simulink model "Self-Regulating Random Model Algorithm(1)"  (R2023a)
settings: Solver=VariableStepAuto  StartTime=0.0  StopTime=20  RelTol=1e-3
libraries: simulink x63, spspowerguiLib x1
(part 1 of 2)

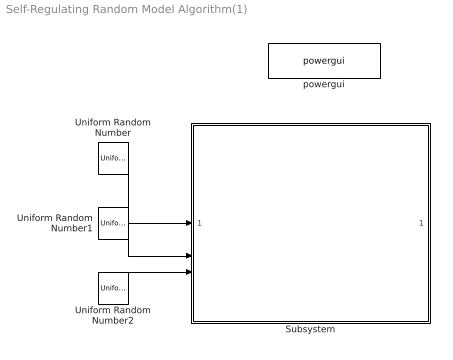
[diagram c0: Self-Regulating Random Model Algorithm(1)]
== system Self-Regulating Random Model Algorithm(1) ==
  Subsystem : Subsystem
  Uniform Random Number : UniformRandomNumber  Minimum=0  Seed=1111  SampleTime=1e-4
  Uniform Random Number1 : UniformRandomNumber  Minimum=0  Seed=3232  SampleTime=1e-4
  Uniform Random Number2 : UniformRandomNumber  Minimum=0  Seed=5566  SampleTime=1e-4
  powergui : spspowerguiLib/powergui  Priority=1  SimulationMode=Discrete  SampleTime=1e-4  frequency=60  Iterations=50  frequencyindice=0  Pbase=100e6  ErrMax=1e-4  UnitsV=kV  UnitsW=MW  buscounter=0  FunctionMessages=off  echomessages=off  EnableUseOfTLC=off  CurrentSourceSwitches=off  DisableSnubberDevices=off  DisableRonSwitches=off  DisableVfSwitches=off  DisplayEquations=off  AutomaticDiscreteSolvers=off  SolverType=Tustin  Interpol=off  ExternalGateDelay=off  methode=off  Ts=0  x0status=blocks  SPID=off  SwTol=0  HookPort=off  NonlinearTolerance=1e-4  nMaxIteration=100  ContinueOnMaxIteration=off  RestoreLinks=warning  ResistiveCurrentMeasurement=off  Frange=[0:2:500]  Ylog=off  Xlog=on  ShowGrid=off  save=off  variable=ZData  structure=sco_motor_wr  ZoomFFT=off  StartTime=4  cycles=75  DisplayStyle=5  fundamental=40  FreqAxis=off  MaxFrequency=300  frequencyindicesteady=1  RmsSteady=1  display=off
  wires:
  Uniform Random Number2/1 -> Subsystem/3(Random_num_add)
  Uniform Random Number1/1 -> Subsystem/2(Random_num_adc)
  Uniform Random Number/1 -> Subsystem/1(Random_num_select)
  Subsystem/1(injection_num) -> ?  "inj_num"

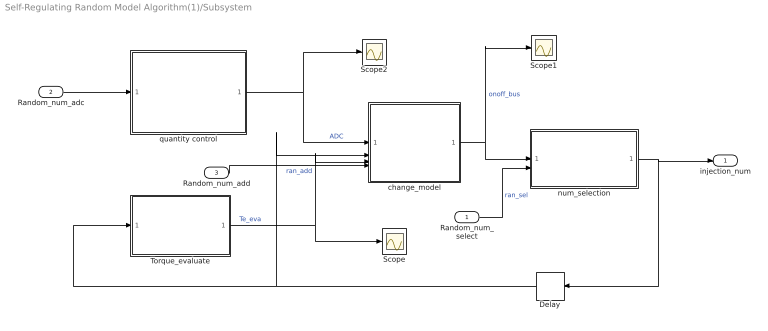
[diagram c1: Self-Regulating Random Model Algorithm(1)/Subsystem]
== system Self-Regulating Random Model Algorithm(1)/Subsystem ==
  Random_num_select : Inport
  Random_num_adc : Inport  Port=2
  Random_num_add : Inport  Port=3
  Delay : Delay  DelayLength=1  InitialCondition=2
  Scope : Scope
  Scope1 : Scope
  Scope2 : Scope
  Torque_evaluate : Subsystem
  change_model : Subsystem
  num_selection : Subsystem
  quantity control : Subsystem
  injection_num : Outport
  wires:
  change_model/1(on/off_signal) -> Scope1/1, num_selection/1(on/off_signal)  "onoff_bus"
  Torque_evaluate/1(Te_eva) -> change_model/3(Te_eva), Scope/1  "Te_eva"
  quantity control/1(A/D/C_operation) -> Scope2/1, change_model/1(A/D/C)  "ADC"
  Delay/1 -> change_model/2(last_num), Torque_evaluate/1(injection_num)
  Random_num_select/1 -> num_selection/2(Random_num)  "ran_sel"
  num_selection/1(injection_num) -> injection_num/1, Delay/1
  Random_num_adc/1 -> quantity control/1(Random_num)
  Random_num_add/1 -> change_model/4(Random_num)  "ran_add"

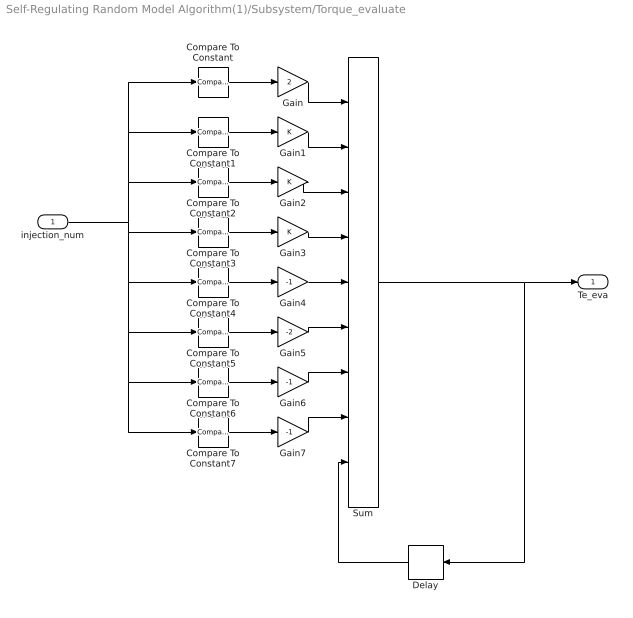
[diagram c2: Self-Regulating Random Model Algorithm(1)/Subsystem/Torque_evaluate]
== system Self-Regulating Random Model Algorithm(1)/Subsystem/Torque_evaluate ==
  injection_num : Inport
  Compare To Constant : simulink/Logic and Bit Operations/Compare To Constant  relop===  const=1  OutDataTypeStr=boolean
  Compare To Constant1 : simulink/Logic and Bit Operations/Compare To Constant  relop===  const=2  OutDataTypeStr=boolean
  Compare To Constant2 : simulink/Logic and Bit Operations/Compare To Constant  relop===  const=8  OutDataTypeStr=boolean
  Compare To Constant3 : simulink/Logic and Bit Operations/Compare To Constant  relop===  const=9  OutDataTypeStr=boolean
  Compare To Constant4 : simulink/Logic and Bit Operations/Compare To Constant  relop===  const=4  OutDataTypeStr=boolean
  Compare To Constant5 : simulink/Logic and Bit Operations/Compare To Constant  relop===  const=5  OutDataTypeStr=boolean
  Compare To Constant6 : simulink/Logic and Bit Operations/Compare To Constant  relop===  const=6  OutDataTypeStr=boolean
  Compare To Constant7 : simulink/Logic and Bit Operations/Compare To Constant  relop===  const=11  OutDataTypeStr=boolean
  Delay : Delay  DelayLength=1  InitialCondition=0
  Gain : Gain  Gain=2  OutDataTypeStr=single
  Gain1 : Gain  OutDataTypeStr=single
  Gain2 : Gain  OutDataTypeStr=single
  Gain3 : Gain  OutDataTypeStr=single
  Gain4 : Gain  Gain=-1  OutDataTypeStr=single
  Gain5 : Gain  Gain=-2  OutDataTypeStr=single
  Gain6 : Gain  Gain=-1  OutDataTypeStr=single
  Gain7 : Gain  Gain=-1  OutDataTypeStr=single
  Sum : Sum  Inputs=+++++++++
  Te_eva : Outport
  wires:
  injection_num/1 -> Compare To Constant5/1, Compare To Constant6/1, Compare To Constant7/1, Compare To Constant4/1, Compare To Constant3/1, Compare To Constant1/1, Compare To Constant/1, Compare To Constant2/1
  Compare To Constant/1 -> Gain/1
  Compare To Constant1/1 -> Gain1/1
  Compare To Constant2/1 -> Gain2/1
  Compare To Constant3/1 -> Gain3/1
  Compare To Constant4/1 -> Gain4/1
  Compare To Constant5/1 -> Gain5/1
  Gain5/1 -> Sum/6
  Gain4/1 -> Sum/5
  Gain3/1 -> Sum/4
  Gain2/1 -> Sum/3
  Gain1/1 -> Sum/2
  Gain/1 -> Sum/1
  Sum/1 -> Delay/1, Te_eva/1
  Delay/1 -> Sum/9
  Compare To Constant7/1 -> Gain7/1
  Gain6/1 -> Sum/7
  Gain7/1 -> Sum/8
  Compare To Constant6/1 -> Gain6/1

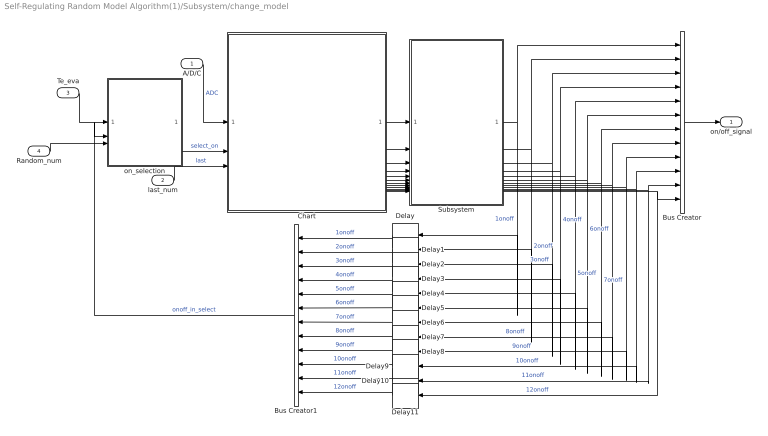
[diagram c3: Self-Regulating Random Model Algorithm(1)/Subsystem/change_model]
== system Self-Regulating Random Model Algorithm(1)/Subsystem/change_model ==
  A/D/C : Inport
  last_num : Inport  Port=2
  Te_eva : Inport  Port=3
  Random_num : Inport  Port=4
  Bus Creator : BusCreator  Inputs=12
  Bus Creator1 : BusCreator  Inputs=12
  Chart : Stateflow chart  TreatAsAtomicUnit=on
  Delay{,1,3..5,7} (6 alike) : Delay  DelayLength=1  InitialCondition=1
  Delay{2,6,8..11} (6 alike) : Delay  DelayLength=1  InitialCondition=0
  Subsystem : Subsystem
  on_selection : Subsystem
  on/off_signal : Outport
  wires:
  Subsystem/5(Condition5) -> Delay4/1, Bus Creator/5  "5onoff"
  Subsystem/6(Condition6) -> Delay5/1, Bus Creator/6  "6onoff"
  Subsystem/7(Condition7) -> Delay6/1, Bus Creator/7  "7onoff"
  Subsystem/8(Condition8) -> Bus Creator/8, Delay7/1  "8onoff"
  Subsystem/9(Condition9) -> Delay8/1, Bus Creator/9  "9onoff"
  Subsystem/10(Condition10) -> Delay9/1, Bus Creator/10  "10onoff"
  Subsystem/11(Condition11) -> Bus Creator/11, Delay10/1  "11onoff"
  Subsystem/12(Condition12) -> Bus Creator/12, Delay11/1  "12onoff"
  Subsystem/1(Condition1) -> Bus Creator/1, Delay/1  "1onoff"
  Subsystem/2(Condition2) -> Bus Creator/2, Delay1/1  "2onoff"
  Subsystem/3(Condition3) -> Delay2/1, Bus Creator/3  "3onoff"
  Subsystem/4(Condition4) -> Delay3/1, Bus Creator/4  "4onoff"
  Bus Creator/1 -> on/off_signal/1
  Te_eva/1 -> on_selection/1(Te_eva)
  Random_num/1 -> on_selection/3(Random_num2)
  Chart/1(Trigger1) -> Subsystem/1(Trigger1)
  Chart/2(Trigger2) -> Subsystem/2(Trigger2)
  Chart/3(Trigger3) -> Subsystem/3(Trigger3)
  Chart/4(Trigger4) -> Subsystem/4(Trigger4)
  Chart/5(Trigger5) -> Subsystem/5(Trigger5)
  Chart/6(Trigger6) -> Subsystem/6(Trigger6)
  Chart/7(Trigger7) -> Subsystem/7(Trigger7)
  Chart/8(Trigger8) -> Subsystem/8(Trigger8)
  Chart/9(Trigger9) -> Subsystem/9(Trigger9)
  Chart/10(Trigger10) -> Subsystem/10(Trigger10)
  Chart/11(Trigger11) -> Subsystem/11(Trigger11)
  Chart/12(Trigger12) -> Subsystem/12(Trigger12)
  on_selection/1(select_on_num) -> Chart/2(select_on_num)  "select_on"
  last_num/1 -> Chart/3(last_num)  "last"
  A/D/C/1 -> Chart/1(A_D_C)  "ADC"
  Delay7/1 -> Bus Creator1/8  "8onoff"
  Delay10/1 -> Bus Creator1/11  "11onoff"
  Delay2/1 -> Bus Creator1/3  "3onoff"
  Delay5/1 -> Bus Creator1/6  "6onoff"
  Delay4/1 -> Bus Creator1/5  "5onoff"
  Delay6/1 -> Bus Creator1/7  "7onoff"
  Delay/1 -> Bus Creator1/1  "1onoff"
  Delay11/1 -> Bus Creator1/12  "12onoff"
  Delay1/1 -> Bus Creator1/2  "2onoff"
  Delay9/1 -> Bus Creator1/10  "10onoff"
  Delay3/1 -> Bus Creator1/4  "4onoff"
  Delay8/1 -> Bus Creator1/9  "9onoff"
  Bus Creator1/1 -> on_selection/2(on/off_bus2)  "onoff_in_select"

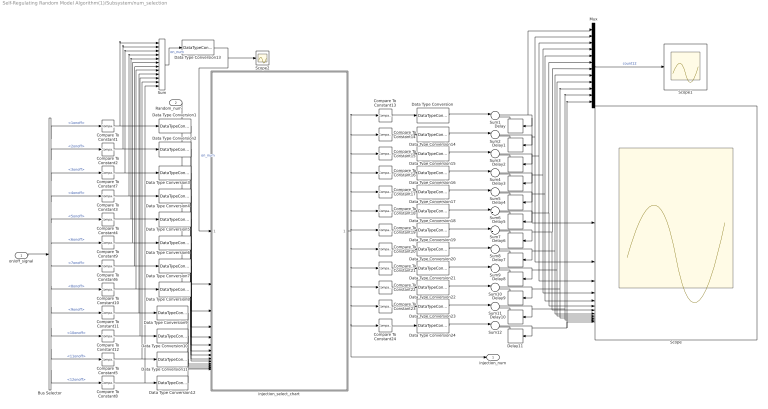
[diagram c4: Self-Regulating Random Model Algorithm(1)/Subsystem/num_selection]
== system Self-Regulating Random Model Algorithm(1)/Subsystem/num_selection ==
  on/off_signal : Inport
  Random_num : Inport  Port=2
  Bus Selector : BusSelector  OutputSignals=1onoff,2onoff,3onoff,4onoff,5onoff,6onoff,7onoff,8onoff,9onoff,10onoff,11onoff,12onoff
  Compare To Constant{1..12} (12 alike) : simulink/Logic and Bit Operations/Compare To Constant  relop===  const=1  OutDataTypeStr=boolean
  Compare To Constant13 : simulink/Logic and Bit Operations/Compare To Constant  relop===  const=1  OutDataTypeStr=uint8
  Compare To Constant14 : simulink/Logic and Bit Operations/Compare To Constant  relop===  const=2  OutDataTypeStr=uint8
  Compare To Constant15 : simulink/Logic and Bit Operations/Compare To Constant  relop===  const=3  OutDataTypeStr=uint8
  Compare To Constant16 : simulink/Logic and Bit Operations/Compare To Constant  relop===  const=4  OutDataTypeStr=uint8
  Compare To Constant17 : simulink/Logic and Bit Operations/Compare To Constant  relop===  const=5  OutDataTypeStr=uint8
  Compare To Constant18 : simulink/Logic and Bit Operations/Compare To Constant  relop===  const=6  OutDataTypeStr=uint8
  Compare To Constant19 : simulink/Logic and Bit Operations/Compare To Constant  relop===  const=7  OutDataTypeStr=uint8
  Compare To Constant20 : simulink/Logic and Bit Operations/Compare To Constant  relop===  const=8  OutDataTypeStr=uint8
  Compare To Constant21 : simulink/Logic and Bit Operations/Compare To Constant  relop===  const=9  OutDataTypeStr=uint8
  Compare To Constant22 : simulink/Logic and Bit Operations/Compare To Constant  relop===  const=10  OutDataTypeStr=uint8
  Compare To Constant23 : simulink/Logic and Bit Operations/Compare To Constant  relop===  const=11  OutDataTypeStr=uint8
  Compare To Constant24 : simulink/Logic and Bit Operations/Compare To Constant  relop===  const=12  OutDataTypeStr=uint8
  Data Type Conversion{,13..24} (13 alike) : DataTypeConversion  OutDataTypeStr=single
  Data Type Conversion{1..12} (12 alike) : DataTypeConversion  OutDataTypeStr=uint8
  Delay{,1..11} (12 alike) : Delay  DelayLength=1  InitialCondition=0
  Mux : Mux  Inputs=12
  Scope : Scope  NumInputPorts=12
  Scope1 : Scope
  Scope2 : Scope
  Sum : Sum  Inputs=++++++++++++
  Sum{1..12} (12 alike) : Sum  Inputs=|++
  injection_select_chart : Stateflow chart  TreatAsAtomicUnit=on
  injection_num : Outport
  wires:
  Bus Selector/11 -> Compare To Constant5/1  "<11onoff>"
  Bus Selector/7 -> Compare To Constant6/1  "<7onoff>"
  Bus Selector/3 -> Compare To Constant7/1  "<3onoff>"
  Bus Selector/2 -> Compare To Constant2/1  "<2onoff>"
  on/off_signal/1 -> Bus Selector/1
  Bus Selector/6 -> Compare To Constant9/1  "<6onoff>"
  Bus Selector/5 -> Compare To Constant4/1  "<5onoff>"
  Bus Selector/1 -> Compare To Constant1/1  "<1onoff>"
  Bus Selector/8 -> Compare To Constant10/1  "<8onoff>"
  Bus Selector/9 -> Compare To Constant11/1  "<9onoff>"
  Bus Selector/4 -> Compare To Constant3/1  "<4onoff>"
  Bus Selector/10 -> Compare To Constant12/1  "<10onoff>"
  Bus Selector/12 -> Compare To Constant8/1  "<12onoff>"
  Compare To Constant1/1 -> Sum/1, Data Type Conversion1/1
  Compare To Constant2/1 -> Data Type Conversion2/1, Sum/2
  Compare To Constant3/1 -> Sum/4, Data Type Conversion4/1
  Compare To Constant9/1 -> Sum/6, Data Type Conversion6/1
  Compare To Constant4/1 -> Sum/5, Data Type Conversion5/1
  Compare To Constant10/1 -> Sum/8, Data Type Conversion8/1
  Compare To Constant12/1 -> Sum/10, Data Type Conversion10/1
  Compare To Constant11/1 -> Sum/9, Data Type Conversion9/1
  Compare To Constant8/1 -> Sum/12, Data Type Conversion12/1
  Compare To Constant7/1 -> Sum/3, Data Type Conversion3/1
  Compare To Constant6/1 -> Sum/7, Data Type Conversion7/1
  Compare To Constant5/1 -> Sum/11, Data Type Conversion11/1
  Random_num/1 -> injection_select_chart/2(Random_num)
  Data Type Conversion13/1 -> Scope2/1, injection_select_chart/1(On_num)  "on_num"
  injection_select_chart/1(Injection_num) -> Compare To Constant19/1, Compare To Constant18/1, Compare To Constant17/1, Compare To Constant16/1, Compare To Constant15/1, Compare To Constant14/1, Compare To Constant13/1, Compare To Constant20/1, Compare To Constant21/1, Compare To Constant22/1, Compare To Constant23/1, Compare To Constant24/1, injection_num/1
  Data Type Conversion1/1 -> injection_select_chart/3(oo1)
  Data Type Conversion2/1 -> injection_select_chart/4(oo2)
  Data Type Conversion3/1 -> injection_select_chart/5(oo3)
  Data Type Conversion4/1 -> injection_select_chart/6(oo4)
  Data Type Conversion5/1 -> injection_select_chart/7(oo5)
  Data Type Conversion6/1 -> injection_select_chart/8(oo6)
  Data Type Conversion7/1 -> injection_select_chart/9(oo7)
  Data Type Conversion8/1 -> injection_select_chart/10(oo8)
  Data Type Conversion9/1 -> injection_select_chart/11(oo9)
  Data Type Conversion10/1 -> injection_select_chart/12(oo10)
  Data Type Conversion11/1 -> injection_select_chart/13(oo11)
  Data Type Conversion12/1 -> injection_select_chart/14(oo12)
  Sum/1 -> Data Type Conversion13/1  "on_num"
  Sum1/1 -> Mux/1, Delay/1, Scope/1
  Compare To Constant13/1 -> Data Type Conversion/1
  Delay/1 -> Sum1/2
  Delay1/1 -> Sum2/2
  Sum2/1 -> Delay1/1, Mux/2, Scope/2
  Compare To Constant14/1 -> Data Type Conversion14/1
  Delay2/1 -> Sum3/2
  Sum3/1 -> Delay2/1, Mux/3, Scope/3
  Compare To Constant15/1 -> Data Type Conversion15/1
  Delay3/1 -> Sum4/2
  Sum4/1 -> Delay3/1, Mux/4, Scope/4
  Compare To Constant16/1 -> Data Type Conversion16/1
  Delay4/1 -> Sum5/2
  Sum5/1 -> Delay4/1, Mux/5, Scope/5
  Compare To Constant17/1 -> Data Type Conversion17/1
  Delay5/1 -> Sum6/2
  Sum6/1 -> Delay5/1, Mux/6, Scope/6
  Compare To Constant18/1 -> Data Type Conversion18/1
  Delay6/1 -> Sum7/2
  Sum7/1 -> Delay6/1, Mux/7, Scope/7
  Compare To Constant19/1 -> Data Type Conversion19/1
  Delay7/1 -> Sum8/2
  Sum8/1 -> Delay7/1, Mux/8, Scope/8
  Compare To Constant20/1 -> Data Type Conversion20/1
  Delay8/1 -> Sum9/2
  Sum9/1 -> Delay8/1, Mux/9, Scope/9
  Compare To Constant21/1 -> Data Type Conversion21/1
  Delay9/1 -> Sum10/2
  Sum10/1 -> Delay9/1, Mux/10, Scope/10
  Compare To Constant22/1 -> Data Type Conversion22/1
  Delay10/1 -> Sum11/2
  Sum11/1 -> Delay10/1, Mux/11, Scope/11
  Compare To Constant23/1 -> Data Type Conversion23/1
  Delay11/1 -> Sum12/2
  Sum12/1 -> Delay11/1, Mux/12, Scope/12
  Compare To Constant24/1 -> Data Type Conversion24/1
  Data Type Conversion/1 -> Sum1/1
  Data Type Conversion14/1 -> Sum2/1
  Data Type Conversion15/1 -> Sum3/1
  Data Type Conversion16/1 -> Sum4/1
  Data Type Conversion17/1 -> Sum5/1
  Data Type Conversion18/1 -> Sum6/1
  Data Type Conversion19/1 -> Sum7/1
  Data Type Conversion20/1 -> Sum8/1
  Data Type Conversion21/1 -> Sum9/1
  Data Type Conversion22/1 -> Sum10/1
  Data Type Conversion23/1 -> Sum11/1
  Data Type Conversion24/1 -> Sum12/1
  Mux/1 -> Scope1/1  "count12"

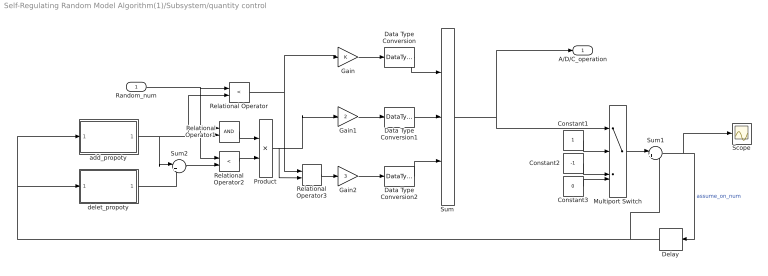
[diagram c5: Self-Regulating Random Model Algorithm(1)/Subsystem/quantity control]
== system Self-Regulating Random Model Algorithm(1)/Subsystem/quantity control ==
  Random_num : Inport
  Constant1 : Constant  OutDataTypeStr=single
  Constant2 : Constant  Value=-1  OutDataTypeStr=single
  Constant3 : Constant  Value=0  OutDataTypeStr=single
  Data Type Conversion : DataTypeConversion  OutDataTypeStr=uint16
  Data Type Conversion1 : DataTypeConversion  OutDataTypeStr=uint16
  Data Type Conversion2 : DataTypeConversion  OutDataTypeStr=uint16
  Delay : Delay  DelayLength=1  InitialCondition=7
  Gain : Gain
  Gain1 : Gain  Gain=2
  Gain2 : Gain  Gain=3
  Multiport Switch : MultiPortSwitch  DiagnosticForDefault=None
  Product : Product
  Relational Operator : RelationalOperator  Operator=<  OutDataTypeStr=boolean
  Relational Operator1 : RelationalOperator  OutDataTypeStr=boolean
  Relational Operator2 : RelationalOperator  Operator=<  OutDataTypeStr=boolean
  Relational Operator3 : RelationalOperator  Operator===  OutDataTypeStr=boolean
  Scope : Scope
  Sum : Sum  Inputs=+++
  Sum1 : Sum  Inputs=|++
  Sum2 : Sum  Inputs=|++
  add_propoty : Subsystem
  delet_propoty : Subsystem
  A/D/C_operation : Outport
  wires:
  Delay/1 -> Sum1/2, delet_propoty/1(Qtt), add_propoty/1(Qtt)
  Gain2/1 -> Data Type Conversion2/1
  Data Type Conversion2/1 -> Sum/3
  Data Type Conversion1/1 -> Sum/2
  Data Type Conversion/1 -> Sum/1
  Gain1/1 -> Data Type Conversion1/1
  Gain/1 -> Data Type Conversion/1
  Random_num/1 -> Relational Operator2/1, Relational Operator1/1, Relational Operator/1
  add_propoty/1(Ppt) -> Sum2/1, Relational Operator1/2, Relational Operator/2
  Relational Operator/1 -> Relational Operator3/1, Gain/1
  Relational Operator1/1 -> Product/1
  Relational Operator2/1 -> Product/2
  Product/1 -> Relational Operator3/2, Gain1/1
  Relational Operator3/1 -> Gain2/1
  Constant1/1 -> Multiport Switch/2
  Constant2/1 -> Multiport Switch/3
  Constant3/1 -> Multiport Switch/4
  Multiport Switch/1 -> Sum1/1
  Sum1/1 -> Scope/1, Delay/1  "assume_on_num"
  Sum2/1 -> Relational Operator2/2
  delet_propoty/1(Ppt) -> Sum2/2
  Sum/1 -> A/D/C_operation/1, Multiport Switch/1

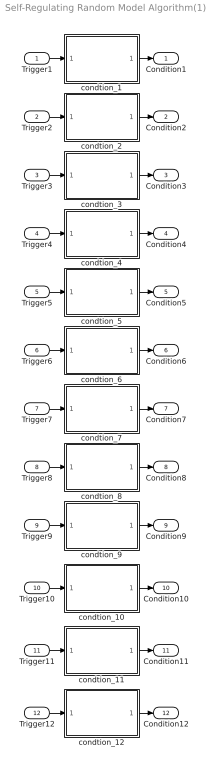
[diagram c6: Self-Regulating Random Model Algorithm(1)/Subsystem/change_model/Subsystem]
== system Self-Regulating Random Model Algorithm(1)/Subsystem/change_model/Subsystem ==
  Trigger1 : Inport
  Trigger2 : Inport  Port=2
  Trigger3 : Inport  Port=3
  Trigger4 : Inport  Port=4
  Trigger5 : Inport  Port=5
  Trigger6 : Inport  Port=6
  Trigger7 : Inport  Port=7
  Trigger8 : Inport  Port=8
  Trigger9 : Inport  Port=9
  Trigger10 : Inport  Port=10
  Trigger11 : Inport  Port=11
  Trigger12 : Inport  Port=12
  condtion_1 : Subsystem
  condtion_10 : Subsystem
  condtion_11 : Subsystem
  condtion_12 : Subsystem
  condtion_2 : Subsystem
  condtion_3 : Subsystem
  condtion_4 : Subsystem
  condtion_5 : Subsystem
  condtion_6 : Subsystem
  condtion_7 : Subsystem
  condtion_8 : Subsystem
  condtion_9 : Subsystem
  Condition1 : Outport
  Condition2 : Outport  Port=2
  Condition3 : Outport  Port=3
  Condition4 : Outport  Port=4
  Condition5 : Outport  Port=5
  Condition6 : Outport  Port=6
  Condition7 : Outport  Port=7
  Condition8 : Outport  Port=8
  Condition9 : Outport  Port=9
  Condition10 : Outport  Port=10
  Condition11 : Outport  Port=11
  Condition12 : Outport  Port=12
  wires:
  Trigger12/1 -> condtion_12/1(Trigger)
  condtion_11/1(Condition) -> Condition11/1
  condtion_3/1(Condition) -> Condition3/1
  condtion_4/1(Condition) -> Condition4/1
  Trigger3/1 -> condtion_3/1(Trigger)
  Trigger11/1 -> condtion_11/1(Trigger)
  Trigger5/1 -> condtion_5/1(Trigger)
  Trigger8/1 -> condtion_8/1(Trigger)
  Trigger6/1 -> condtion_6/1(Trigger)
  condtion_5/1(Condition) -> Condition5/1
  Trigger4/1 -> condtion_4/1(Trigger)
  Trigger9/1 -> condtion_9/1(Trigger)
  condtion_9/1(Condition) -> Condition9/1
  Trigger10/1 -> condtion_10/1(Trigger)
  condtion_6/1(Condition) -> Condition6/1
  condtion_10/1(Condition) -> Condition10/1
  Trigger2/1 -> condtion_2/1(Trigger)
  condtion_2/1(Condition) -> Condition2/1
  Trigger1/1 -> condtion_1/1(Trigger)
  condtion_1/1(Condition) -> Condition1/1
  condtion_12/1(Condition) -> Condition12/1
  Trigger7/1 -> condtion_7/1(Trigger)
  condtion_7/1(Condition) -> Condition7/1
  condtion_8/1(Condition) -> Condition8/1

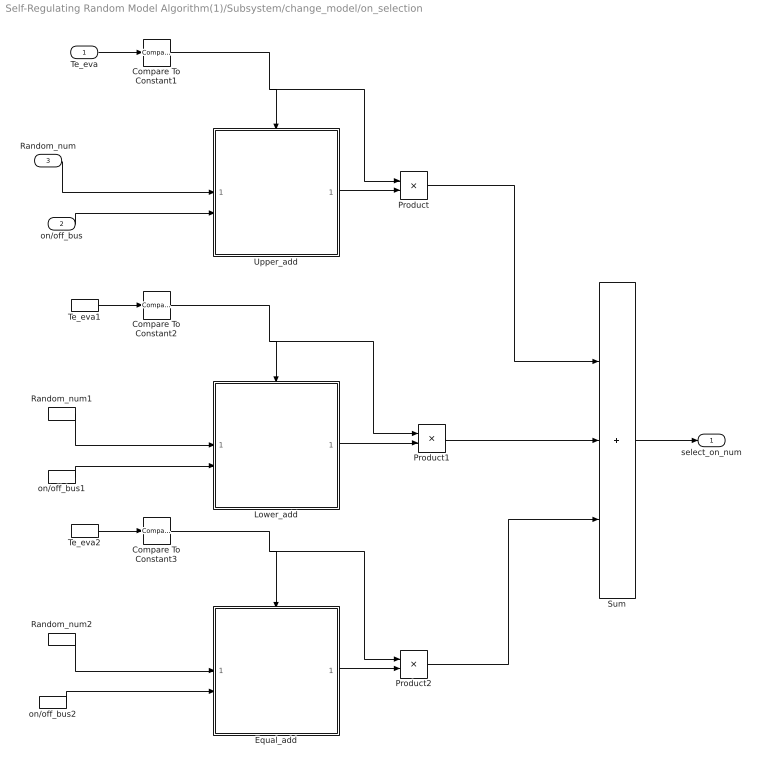
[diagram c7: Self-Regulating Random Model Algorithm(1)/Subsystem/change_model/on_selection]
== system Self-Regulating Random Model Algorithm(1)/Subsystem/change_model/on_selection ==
  Te_eva : Inport
  on/off_bus : Inport  Port=2
  Random_num : Inport  Port=3
  Compare To Constant1 : simulink/Logic and Bit Operations/Compare To Constant  relop=>  const=0  OutDataTypeStr=boolean
  Compare To Constant2 : simulink/Logic and Bit Operations/Compare To Constant  relop=<  const=0  OutDataTypeStr=boolean
  Compare To Constant3 : simulink/Logic and Bit Operations/Compare To Constant  relop===  const=0  OutDataTypeStr=boolean
  Equal_add : Subsystem
  Lower_add : Subsystem
  Product : Product
  Product1 : Product
  Product2 : Product
  Random_num1 : InportShadow  Port=3
  Random_num2 : InportShadow  Port=3
  Sum : Sum  Inputs=+++
  Te_eva1 : InportShadow
  Te_eva2 : InportShadow
  Upper_add : Subsystem
  on/off_bus1 : InportShadow  Port=2
  on/off_bus2 : InportShadow  Port=2
  select_on_num : Outport
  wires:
  Te_eva/1 -> Compare To Constant1/1
  on/off_bus/1 -> Upper_add/2(on/off_bus)
  Random_num/1 -> Upper_add/1(Random_num)
  Compare To Constant1/1 -> Product/1, Upper_add/Enable
  Compare To Constant2/1 -> Product1/1, Lower_add/Enable
  on/off_bus1/1 -> Lower_add/2(on/off_bus)
  Te_eva1/1 -> Compare To Constant2/1
  Random_num1/1 -> Lower_add/1(Random_num)
  Compare To Constant3/1 -> Product2/1, Equal_add/Enable
  Random_num2/1 -> Equal_add/1(Random_num)
  Te_eva2/1 -> Compare To Constant3/1
  on/off_bus2/1 -> Equal_add/2(on/off_bus)
  Upper_add/1(Upper_add_num) -> Product/2
  Product/1 -> Sum/1
  Lower_add/1(Lower_add_num) -> Product1/2
  Product1/1 -> Sum/2
  Equal_add/1(Equal_add_num) -> Product2/2
  Product2/1 -> Sum/3
  Sum/1 -> select_on_num/1

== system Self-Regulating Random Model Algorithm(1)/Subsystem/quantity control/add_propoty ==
  Qtt : Inport
  Constant6 : Constant  Value=7  OutDataTypeStr=single
  Gain : Gain  Gain=0.125
  Sum : Sum  Inputs=|+-
  Ppt : Outport
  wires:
  Constant6/1 -> Sum/1
  Qtt/1 -> Sum/2
  Sum/1 -> Gain/1
  Gain/1 -> Ppt/1

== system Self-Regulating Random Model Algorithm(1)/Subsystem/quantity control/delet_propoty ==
  Qtt : Inport
  Constant6 : Constant  Value=3  OutDataTypeStr=single
  Gain : Gain  Gain=0.125
  Sum : Sum  Inputs=|+-
  Ppt : Outport
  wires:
  Sum/1 -> Gain/1
  Gain/1 -> Ppt/1
  Qtt/1 -> Sum/1
  Constant6/1 -> Sum/2

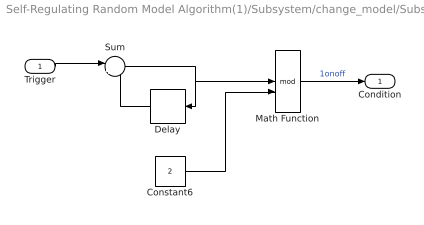
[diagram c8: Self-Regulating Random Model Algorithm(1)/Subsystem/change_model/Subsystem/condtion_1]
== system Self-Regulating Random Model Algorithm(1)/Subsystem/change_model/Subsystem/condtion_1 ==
  Trigger : Inport
  Constant6 : Constant  Value=2  OutDataTypeStr=single
  Delay : Delay  DelayLength=1  InitialCondition=1
  Math Function : Math  Operator=mod  SignedPower=on
  Sum : Sum  Inputs=|++
  Condition : Outport
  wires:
  Constant6/1 -> Math Function/2
  Math Function/1 -> Condition/1  "1onoff"
  Trigger/1 -> Sum/1
  Delay/1 -> Sum/2
  Sum/1 -> Delay/1, Math Function/1

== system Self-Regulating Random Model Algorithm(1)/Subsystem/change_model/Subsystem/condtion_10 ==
  Trigger : Inport
  Constant6 : Constant  Value=2  OutDataTypeStr=single
  Delay : Delay  DelayLength=1  InitialCondition=0
  Math Function : Math  Operator=mod  SignedPower=on
  Sum : Sum  Inputs=|++
  Condition : Outport
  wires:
  Constant6/1 -> Math Function/2
  Math Function/1 -> Condition/1
  Trigger/1 -> Sum/1
  Delay/1 -> Sum/2
  Sum/1 -> Delay/1, Math Function/1

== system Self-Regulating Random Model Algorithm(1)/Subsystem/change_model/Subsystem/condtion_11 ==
  Trigger : Inport
  Constant6 : Constant  Value=2  OutDataTypeStr=single
  Delay : Delay  DelayLength=1  InitialCondition=0
  Math Function : Math  Operator=mod  SignedPower=on
  Sum : Sum  Inputs=|++
  Condition : Outport
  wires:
  Constant6/1 -> Math Function/2
  Math Function/1 -> Condition/1
  Trigger/1 -> Sum/1
  Delay/1 -> Sum/2
  Sum/1 -> Delay/1, Math Function/1

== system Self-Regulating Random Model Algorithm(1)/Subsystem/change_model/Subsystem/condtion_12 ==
  Trigger : Inport
  Constant6 : Constant  Value=2  OutDataTypeStr=single
  Delay : Delay  DelayLength=1  InitialCondition=0
  Math Function : Math  Operator=mod  SignedPower=on
  Sum : Sum  Inputs=|++
  Condition : Outport
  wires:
  Constant6/1 -> Math Function/2
  Math Function/1 -> Condition/1
  Trigger/1 -> Sum/1
  Delay/1 -> Sum/2
  Sum/1 -> Delay/1, Math Function/1

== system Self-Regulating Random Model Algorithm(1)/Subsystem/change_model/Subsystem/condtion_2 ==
  Trigger : Inport
  Constant6 : Constant  Value=2  OutDataTypeStr=single
  Delay : Delay  DelayLength=1  InitialCondition=1
  Math Function : Math  Operator=mod  SignedPower=on
  Sum : Sum  Inputs=|++
  Condition : Outport
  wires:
  Constant6/1 -> Math Function/2
  Math Function/1 -> Condition/1
  Trigger/1 -> Sum/1
  Delay/1 -> Sum/2
  Sum/1 -> Delay/1, Math Function/1

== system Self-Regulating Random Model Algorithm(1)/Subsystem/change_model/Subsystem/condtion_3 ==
  Trigger : Inport
  Constant6 : Constant  Value=2  OutDataTypeStr=single
  Delay : Delay  DelayLength=1  InitialCondition=1
  Math Function : Math  Operator=mod  SignedPower=on
  Sum : Sum  Inputs=|++
  Condition : Outport
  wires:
  Constant6/1 -> Math Function/2
  Math Function/1 -> Condition/1
  Trigger/1 -> Sum/1
  Delay/1 -> Sum/2
  Sum/1 -> Delay/1, Math Function/1

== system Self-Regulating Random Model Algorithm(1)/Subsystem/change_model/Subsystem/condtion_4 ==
  Trigger : Inport
  Constant6 : Constant  Value=2  OutDataTypeStr=single
  Delay : Delay  DelayLength=1  InitialCondition=1
  Math Function : Math  Operator=mod  SignedPower=on
  Sum : Sum  Inputs=|++
  Condition : Outport
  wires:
  Constant6/1 -> Math Function/2
  Math Function/1 -> Condition/1
  Trigger/1 -> Sum/1
  Delay/1 -> Sum/2
  Sum/1 -> Delay/1, Math Function/1

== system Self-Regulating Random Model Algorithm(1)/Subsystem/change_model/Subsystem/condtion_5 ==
  Trigger : Inport
  Constant6 : Constant  Value=2  OutDataTypeStr=single
  Delay : Delay  DelayLength=1  InitialCondition=1
  Math Function : Math  Operator=mod  SignedPower=on
  Sum : Sum  Inputs=|++
  Condition : Outport
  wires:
  Constant6/1 -> Math Function/2
  Math Function/1 -> Condition/1
  Trigger/1 -> Sum/1
  Delay/1 -> Sum/2
  Sum/1 -> Delay/1, Math Function/1

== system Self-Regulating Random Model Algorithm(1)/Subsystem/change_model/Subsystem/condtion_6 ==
  Trigger : Inport
  Constant6 : Constant  Value=2  OutDataTypeStr=single
  Delay : Delay  DelayLength=1  InitialCondition=1
  Math Function : Math  Operator=mod  SignedPower=on
  Sum : Sum  Inputs=|++
  Condition : Outport
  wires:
  Constant6/1 -> Math Function/2
  Math Function/1 -> Condition/1
  Trigger/1 -> Sum/1
  Delay/1 -> Sum/2
  Sum/1 -> Delay/1, Math Function/1

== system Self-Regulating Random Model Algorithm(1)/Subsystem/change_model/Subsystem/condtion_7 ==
  Trigger : Inport
  Constant6 : Constant  Value=2  OutDataTypeStr=single
  Delay : Delay  DelayLength=1  InitialCondition=0
  Math Function : Math  Operator=mod  SignedPower=on
  Sum : Sum  Inputs=|++
  Condition : Outport
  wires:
  Constant6/1 -> Math Function/2
  Math Function/1 -> Condition/1
  Trigger/1 -> Sum/1
  Delay/1 -> Sum/2
  Sum/1 -> Delay/1, Math Function/1

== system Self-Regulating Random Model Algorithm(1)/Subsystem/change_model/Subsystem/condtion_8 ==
  Trigger : Inport
  Constant6 : Constant  Value=2  OutDataTypeStr=single
  Delay : Delay  DelayLength=1  InitialCondition=1
  Math Function : Math  Operator=mod  SignedPower=on
  Sum : Sum  Inputs=|++
  Condition : Outport
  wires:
  Constant6/1 -> Math Function/2
  Math Function/1 -> Condition/1
  Trigger/1 -> Sum/1
  Delay/1 -> Sum/2
  Sum/1 -> Delay/1, Math Function/1

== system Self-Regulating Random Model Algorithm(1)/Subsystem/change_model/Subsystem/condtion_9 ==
  Trigger : Inport
  Constant6 : Constant  Value=2  OutDataTypeStr=single
  Delay : Delay  DelayLength=1  InitialCondition=0
  Math Function : Math  Operator=mod  SignedPower=on
  Sum : Sum  Inputs=|++
  Condition : Outport
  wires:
  Constant6/1 -> Math Function/2
  Math Function/1 -> Condition/1
  Trigger/1 -> Sum/1
  Delay/1 -> Sum/2
  Sum/1 -> Delay/1, Math Function/1

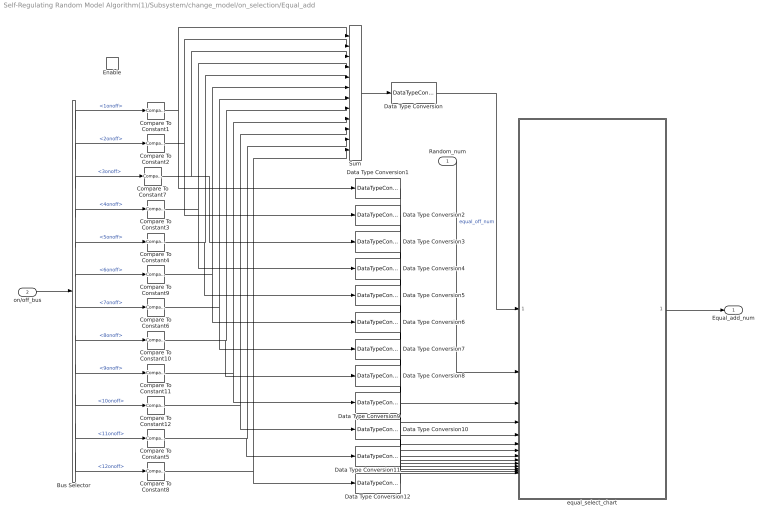
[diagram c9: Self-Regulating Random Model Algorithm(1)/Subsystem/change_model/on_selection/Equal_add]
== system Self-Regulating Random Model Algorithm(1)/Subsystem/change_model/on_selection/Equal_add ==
  Random_num : Inport
  on/off_bus : Inport  Port=2
  Enable : EnablePort  StatesWhenEnabling=reset
  Bus Selector : BusSelector  OutputSignals=1onoff,2onoff,3onoff,4onoff,5onoff,6onoff,7onoff,8onoff,9onoff,10onoff,11onoff,12onoff
  Compare To Constant{1..12} (12 alike) : simulink/Logic and Bit Operations/Compare To Constant  relop===  const=0  OutDataTypeStr=boolean
  Data Type Conversion : DataTypeConversion  OutDataTypeStr=single
  Data Type Conversion{1..12} (12 alike) : DataTypeConversion  OutDataTypeStr=uint8
  Sum : Sum  Inputs=++++++++++++
  equal_select_chart : Stateflow chart  TreatAsAtomicUnit=on
  Equal_add_num : Outport
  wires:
  on/off_bus/1 -> Bus Selector/1
  Bus Selector/1 -> Compare To Constant1/1  "<1onoff>"
  Bus Selector/2 -> Compare To Constant2/1  "<2onoff>"
  Bus Selector/4 -> Compare To Constant3/1  "<4onoff>"
  Bus Selector/12 -> Compare To Constant8/1  "<12onoff>"
  Compare To Constant1/1 -> Data Type Conversion1/1, Sum/1
  Sum/1 -> Data Type Conversion/1
  Compare To Constant2/1 -> Data Type Conversion2/1, Sum/2
  Compare To Constant3/1 -> Data Type Conversion4/1, Sum/4
  Compare To Constant4/1 -> Data Type Conversion5/1, Sum/5
  Compare To Constant9/1 -> Data Type Conversion6/1, Sum/6
  Compare To Constant10/1 -> Data Type Conversion8/1, Sum/8
  Compare To Constant11/1 -> Data Type Conversion9/1, Sum/9
  Compare To Constant12/1 -> Data Type Conversion10/1, Sum/10
  Compare To Constant8/1 -> Sum/12, Data Type Conversion12/1
  Data Type Conversion/1 -> equal_select_chart/1(Off_num)  "equal_off_num"
  Random_num/1 -> equal_select_chart/2(Random_num)
  equal_select_chart/1(Equal_add_num) -> Equal_add_num/1
  Bus Selector/5 -> Compare To Constant4/1  "<5onoff>"
  Bus Selector/6 -> Compare To Constant9/1  "<6onoff>"
  Bus Selector/8 -> Compare To Constant10/1  "<8onoff>"
  Bus Selector/9 -> Compare To Constant11/1  "<9onoff>"
  Bus Selector/10 -> Compare To Constant12/1  "<10onoff>"
  Bus Selector/3 -> Compare To Constant7/1  "<3onoff>"
  Bus Selector/11 -> Compare To Constant5/1  "<11onoff>"
  Bus Selector/7 -> Compare To Constant6/1  "<7onoff>"
  Compare To Constant5/1 -> Data Type Conversion11/1, Sum/11
  Compare To Constant6/1 -> Data Type Conversion7/1, Sum/7
  Compare To Constant7/1 -> Data Type Conversion3/1, Sum/3
  Data Type Conversion1/1 -> equal_select_chart/3(oo1)
  Data Type Conversion2/1 -> equal_select_chart/4(oo2)
  Data Type Conversion3/1 -> equal_select_chart/5(oo3)
  Data Type Conversion4/1 -> equal_select_chart/6(oo4)
  Data Type Conversion5/1 -> equal_select_chart/7(oo5)
  Data Type Conversion6/1 -> equal_select_chart/8(oo6)
  Data Type Conversion7/1 -> equal_select_chart/9(oo7)
  Data Type Conversion8/1 -> equal_select_chart/10(oo8)
  Data Type Conversion9/1 -> equal_select_chart/11(oo9)
  Data Type Conversion10/1 -> equal_select_chart/12(oo10)
  Data Type Conversion11/1 -> equal_select_chart/13(oo11)
  Data Type Conversion12/1 -> equal_select_chart/14(oo12)

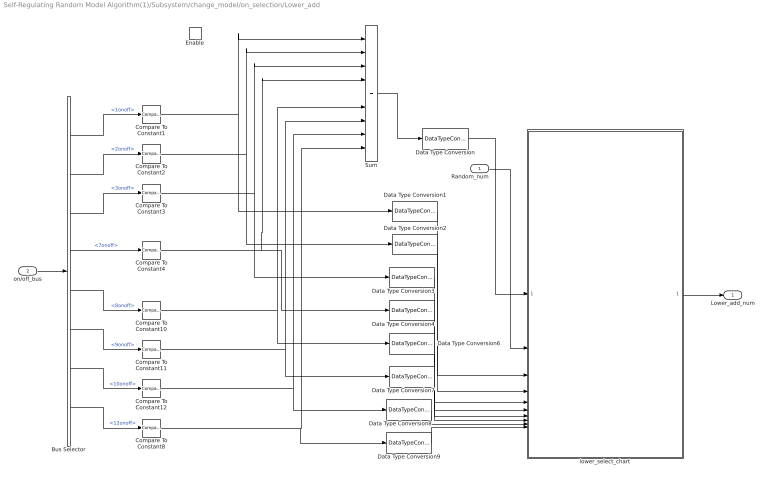
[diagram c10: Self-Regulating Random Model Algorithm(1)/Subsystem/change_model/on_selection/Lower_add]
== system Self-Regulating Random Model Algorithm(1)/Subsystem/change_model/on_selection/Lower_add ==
  Random_num : Inport
  on/off_bus : Inport  Port=2
  Enable : EnablePort  StatesWhenEnabling=reset
  Bus Selector : BusSelector  OutputSignals=1onoff,2onoff,3onoff,7onoff,8onoff,9onoff,10onoff,12onoff
  Compare To Constant{1..4,8,10..12} (8 alike) : simulink/Logic and Bit Operations/Compare To Constant  relop===  const=0  OutDataTypeStr=boolean
  Data Type Conversion : DataTypeConversion  OutDataTypeStr=single
  Data Type Conversion{1..4,6..9} (8 alike) : DataTypeConversion  OutDataTypeStr=uint8
  Sum : Sum  Inputs=+++++++++
  lower_select_chart : Stateflow chart  TreatAsAtomicUnit=on
  Lower_add_num : Outport
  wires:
  on/off_bus/1 -> Bus Selector/1
  Bus Selector/1 -> Compare To Constant1/1  "<1onoff>"
  Bus Selector/2 -> Compare To Constant2/1  "<2onoff>"
  Bus Selector/3 -> Compare To Constant3/1  "<3onoff>"
  Bus Selector/8 -> Compare To Constant8/1  "<12onoff>"
  Compare To Constant1/1 -> Data Type Conversion1/1, Sum/1
  Sum/1 -> Data Type Conversion/1
  Compare To Constant2/1 -> Data Type Conversion2/1, Sum/2
  Compare To Constant3/1 -> Data Type Conversion3/1, Sum/3
  Compare To Constant4/1 -> Sum/4, Data Type Conversion4/1
  Compare To Constant10/1 -> Data Type Conversion6/1, Sum/6
  Compare To Constant11/1 -> Data Type Conversion7/1, Sum/7
  Compare To Constant12/1 -> Data Type Conversion8/1, Sum/8
  Compare To Constant8/1 -> Data Type Conversion9/1, Sum/9
  Data Type Conversion/1 -> lower_select_chart/1(Off_num)
  Random_num/1 -> lower_select_chart/2(Random_num)
  lower_select_chart/1(Lower_add_num) -> Lower_add_num/1
  Bus Selector/4 -> Compare To Constant4/1  "<7onoff>"
  Bus Selector/5 -> Compare To Constant10/1  "<8onoff>"
  Bus Selector/6 -> Compare To Constant11/1  "<9onoff>"
  Bus Selector/7 -> Compare To Constant12/1  "<10onoff>"
  Data Type Conversion1/1 -> lower_select_chart/3(oo1)
  Data Type Conversion2/1 -> lower_select_chart/4(oo2)
  Data Type Conversion3/1 -> lower_select_chart/5(oo3)
  Data Type Conversion4/1 -> lower_select_chart/6(oo7)
  Data Type Conversion6/1 -> lower_select_chart/7(oo8)
  Data Type Conversion7/1 -> lower_select_chart/8(oo9)
  Data Type Conversion8/1 -> lower_select_chart/9(oo10)
  Data Type Conversion9/1 -> lower_select_chart/10(oo12)

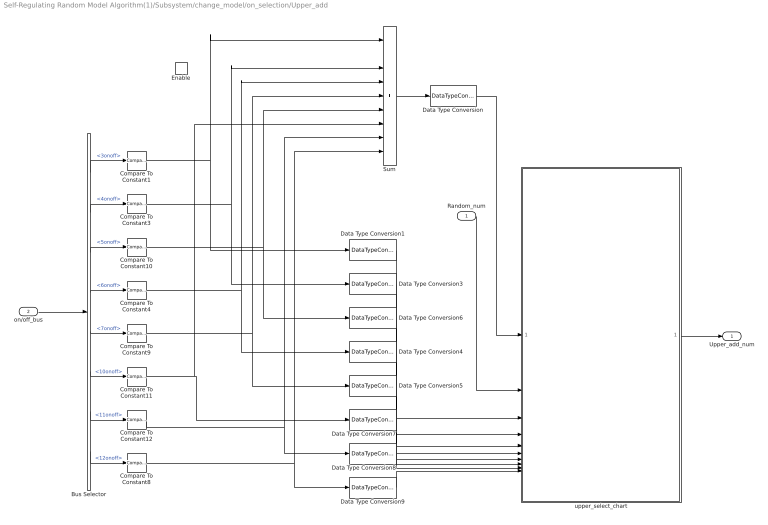
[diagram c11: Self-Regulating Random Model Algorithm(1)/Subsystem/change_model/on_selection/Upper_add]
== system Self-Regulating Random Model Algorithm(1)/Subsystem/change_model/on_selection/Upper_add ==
  Random_num : Inport
  on/off_bus : Inport  Port=2
  Enable : EnablePort  StatesWhenEnabling=reset
  Bus Selector : BusSelector  OutputSignals=3onoff,4onoff,5onoff,6onoff,7onoff,10onoff,11onoff,12onoff
  Compare To Constant{1,3..4,8..12} (8 alike) : simulink/Logic and Bit Operations/Compare To Constant  relop===  const=0  OutDataTypeStr=boolean
  Data Type Conversion : DataTypeConversion  OutDataTypeStr=single
  Data Type Conversion{1,3..9} (8 alike) : DataTypeConversion  OutDataTypeStr=uint8
  Sum : Sum  Inputs=+++++++++
  upper_select_chart : Stateflow chart  TreatAsAtomicUnit=on
  Upper_add_num : Outport
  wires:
  on/off_bus/1 -> Bus Selector/1
  Bus Selector/1 -> Compare To Constant1/1  "<3onoff>"
  Bus Selector/2 -> Compare To Constant3/1  "<4onoff>"
  Bus Selector/4 -> Compare To Constant4/1  "<6onoff>"
  Bus Selector/5 -> Compare To Constant9/1  "<7onoff>"
  Bus Selector/6 -> Compare To Constant11/1  "<10onoff>"
  Bus Selector/7 -> Compare To Constant12/1  "<11onoff>"
  Bus Selector/8 -> Compare To Constant8/1  "<12onoff>"
  Sum/1 -> Data Type Conversion/1
  Compare To Constant3/1 -> Data Type Conversion3/1, Sum/3
  Compare To Constant4/1 -> Sum/4, Data Type Conversion4/1
  Compare To Constant9/1 -> Sum/5, Data Type Conversion5/1
  Compare To Constant10/1 -> Data Type Conversion6/1, Sum/6
  Compare To Constant11/1 -> Sum/7, Data Type Conversion7/1
  Compare To Constant12/1 -> Data Type Conversion8/1, Sum/8
  Compare To Constant8/1 -> Data Type Conversion9/1, Sum/9
  Data Type Conversion/1 -> upper_select_chart/1(Off_num)
  Random_num/1 -> upper_select_chart/2(Random_num)
  upper_select_chart/1(Upper_add_num) -> Upper_add_num/1
  Compare To Constant1/1 -> Sum/1, Data Type Conversion1/1
  Data Type Conversion1/1 -> upper_select_chart/3(oo3)
  Data Type Conversion3/1 -> upper_select_chart/4(oo4)
  Data Type Conversion4/1 -> upper_select_chart/6(oo6)
  Data Type Conversion5/1 -> upper_select_chart/7(oo7)
  Data Type Conversion6/1 -> upper_select_chart/5(oo5)
  Data Type Conversion7/1 -> upper_select_chart/8(oo10)
  Data Type Conversion8/1 -> upper_select_chart/9(oo11)
  Data Type Conversion9/1 -> upper_select_chart/10(oo12)
  Bus Selector/3 -> Compare To Constant10/1  "<5onoff>"

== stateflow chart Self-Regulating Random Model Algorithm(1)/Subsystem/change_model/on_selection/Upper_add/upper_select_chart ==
  state select_num=upper_select(x) [function]
    (default) -> (junction 546)
    (junction 497) -> (junction 500) : {x=x-1}
    (junction 500) -> (junction 498) : [x==0]
    (junction 546) -> (junction 497) : [oo3==1]
    (junction 500) -> (junction 528)
    (junction 498) -> (junction 443) : {select_num=3}
    (junction 546) -> (junction 528)
    (junction 528) -> (junction 563)
    (junction 558) -> (junction 562) : {x=x-1}
    (junction 562) -> (junction 564) : [x==0]
    (junction 563) -> (junction 558) : [oo4==1]
    (junction 562) -> (junction 471)
    (junction 564) -> (junction 508) : {select_num=4}
    (junction 563) -> (junction 471)
    (junction 472) -> (junction 470) : {x=x-1}
    (junction 470) -> (junction 468) : [x==0]
    (junction 471) -> (junction 472) : [oo6==1]
    (junction 470) -> (junction 457)
    (junction 468) -> (junction 454) : {select_num=6}
    (junction 471) -> (junction 457)
    (junction 456) -> (junction 455) : {x=x-1}
    (junction 455) -> (junction 458) : [x==0]
    (junction 457) -> (junction 456) : [oo7==1]
    (junction 455) -> (junction 452)
    (junction 458) -> (junction 453) : {select_num=7}
    (junction 457) -> (junction 452)
    (junction 452) -> (junction 444) : [oo5==1]
    (junction 444) -> (junction 450) : {x=x-1}
    (junction 450) -> (junction 448) : [x==0]
    (junction 450) -> (junction 479)
    (junction 452) -> (junction 479)
    (junction 448) -> (junction 557) : {select_num=5}
    (junction 479) -> (junction 478) : [oo10==1]
    (junction 478) -> (junction 476) : {x=x-1}
    (junction 476) -> (junction 475) : [x==0]
    (junction 476) -> (junction 491)
    (junction 479) -> (junction 491)
    (junction 475) -> (junction 531) : {select_num=10}
    (junction 491) -> (junction 495) : [oo11==1]
    (junction 495) -> (junction 488) : {x=x-1}
    (junction 488) -> (junction 493) : [x==0]
    (junction 488) -> (junction 554)
    (junction 491) -> (junction 554)
    (junction 493) -> (junction 505) : {select_num=11}
    (junction 554) -> (junction 511) : {select_num=12}
    (junction 505) -> (junction 511)
    (junction 531) -> (junction 505)
    (junction 504) -> (junction 531)
    (junction 557) -> (junction 504)
    (junction 454) -> (junction 453)
    (junction 508) -> (junction 454)
    (junction 453) -> (junction 557)
    (junction 513) -> (junction 508)
    (junction 511) -> (junction 487)
    (junction 443) -> (junction 513)
  state upper_add_select_block
    exit:
  (default) -> upper_add_select_block : {upper_check_width = 1/Off_num; upper_step=ceil(Random_num/upper_check_width); Upper_add_num=upper_select(upper_step);}
  upper_add_select_block -> upper_add_select_block : {upper_check_width = 1/Off_num; upper_step=ceil(Random_num/upper_check_width); Upper_add_num=upper_select(upper_step)}
  data: select_num function_output single; x function_input double; Off_num input; Random_num input; Upper_add_num output single; oo3 input; oo4 input; oo5 input; oo6 input; oo7 input; oo10 input; oo11 input; oo12 input; upper_check_width local single; upper_step local single

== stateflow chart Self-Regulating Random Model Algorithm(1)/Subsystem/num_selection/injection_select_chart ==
  state select_num=check_select(x) [function]
    (default) -> (junction 8)
    (junction 13) -> (junction 32) : {x=x-1}
    (junction 32) -> (junction 33) : [x==0]
    (junction 8) -> (junction 13) : [oo1==1]
    (junction 32) -> (junction 44)
    (junction 33) -> (junction 36) : {select_num=1}
    (junction 8) -> (junction 44)
    (junction 38) -> (junction 40) : {x=x-1}
    (junction 40) -> (junction 41) : [x==0]
    (junction 44) -> (junction 38) : [oo2==1]
    (junction 40) -> (junction 54)
    (junction 41) -> (junction 56) : {select_num=2}
    (junction 44) -> (junction 54)
    (junction 48) -> (junction 51) : {x=x-1}
    (junction 51) -> (junction 49) : [x==0]
    (junction 54) -> (junction 48) : [oo3==1]
    (junction 51) -> (junction 60)
    (junction 49) -> (junction 142) : {select_num=3}
    (junction 54) -> (junction 60)
    (junction 61) -> (junction 65) : {x=x-1}
    (junction 65) -> (junction 66) : [x==0]
    (junction 60) -> (junction 61) : [oo4==1]
    (junction 65) -> (junction 79)
    (junction 66) -> (junction 143) : {select_num=4}
    (junction 60) -> (junction 79)
    (junction 80) -> (junction 84) : {x=x-1}
    (junction 84) -> (junction 85) : [x==0]
    (junction 79) -> (junction 80) : [oo5==1]
    (junction 84) -> (junction 96)
    (junction 85) -> (junction 144) : {select_num=5}
    (junction 79) -> (junction 96)
    (junction 94) -> (junction 93) : {x=x-1}
    (junction 93) -> (junction 90) : [x==0]
    (junction 96) -> (junction 94) : [oo6==1]
    (junction 93) -> (junction 105)
    (junction 90) -> (junction 148) : {select_num=6}
    (junction 96) -> (junction 105)
    (junction 103) -> (junction 102) : {x=x-1}
    (junction 102) -> (junction 99) : [x==0]
    (junction 105) -> (junction 103) : [oo7==1]
    (junction 102) -> (junction 114)
    (junction 99) -> (junction 149) : {select_num=7}
    (junction 105) -> (junction 114)
    (junction 114) -> (junction 112) : [oo8==1]
    (junction 112) -> (junction 111) : {x=x-1}
    (junction 111) -> (junction 108) : [x==0]
    (junction 111) -> (junction 123)
    (junction 114) -> (junction 123)
    (junction 108) -> (junction 153) : {select_num=8}
    (junction 123) -> (junction 121) : [oo9==1]
    (junction 121) -> (junction 120) : {x=x-1}
    (junction 120) -> (junction 117) : [x==0]
    (junction 120) -> (junction 132)
    (junction 123) -> (junction 132)
    (junction 117) -> (junction 155) : {select_num=9}
    (junction 132) -> (junction 130) : [oo10==1]
    (junction 130) -> (junction 129) : {x=x-1}
    (junction 129) -> (junction 126) : [x==0]
    (junction 129) -> (junction 141)
    (junction 132) -> (junction 141)
    (junction 126) -> (junction 157) : {select_num=10}
    (junction 141) -> (junction 139) : [oo11==1]
    (junction 139) -> (junction 138) : {x=x-1}
    (junction 138) -> (junction 135) : [x==0]
    (junction 138) -> (junction 161)
    (junction 141) -> (junction 161)
    (junction 135) -> (junction 159) : {select_num=11}
    (junction 161) -> (junction 163) : {select_num=12}
    (junction 159) -> (junction 163)
    (junction 157) -> (junction 159)
    (junction 155) -> (junction 157)
    (junction 36) -> (junction 56)
    (junction 153) -> (junction 155)
    (junction 148) -> (junction 149)
    (junction 144) -> (junction 148)
    (junction 149) -> (junction 153)
    (junction 163) -> (junction 175)
    (junction 143) -> (junction 144)
    (junction 142) -> (junction 143)
    (junction 56) -> (junction 142)
  state injection_select_block
    exit:
  (default) -> injection_select_block : {check_width = 1/On_num; step=ceil(Random_num/check_width); Injection_num=check_select(step);}
  injection_select_block -> injection_select_block : {check_width = 1/On_num; step=ceil(Random_num/check_width); Injection_num=check_select(step)}
  data: select_num function_output single; x function_input single; On_num input; Random_num input; Injection_num output single; oo1 input; oo2 input; oo3 input; oo4 input; oo5 input; oo6 input; oo7 input; oo8 input; oo9 input; oo10 input; oo11 input; oo12 input; check_width local single; step local single

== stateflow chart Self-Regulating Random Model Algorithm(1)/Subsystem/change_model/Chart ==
  state Clear_block
    en:
  (junction 233) -> Clear_block
  Clear_block -> (junction 41) : {Trigger1=0; Trigger2=0; Trigger3=0; Trigger4=0; Trigger5=0; Trigger6=0; Trigger7=0; Trigger8=0; Trigger9=0; Trigger10=0; Trigger11=0; Trigger12=0; }
  (default) -> (junction 41)
  (junction 41) -> (junction 43) : [A_D_C==1||A_D_C==3]
  (junction 43) -> (junction 63)
  (junction 41) -> (junction 43)
  (junction 41) -> (junction 45) : [A_D_C==2]
  (junction 45) -> (junction 183)
  (junction 146) -> (junction 45) : [A_D_C==3]
  (junction 183) -> (junction 182) : [last_num==1]
  (junction 183) -> (junction 185)
  (junction 182) -> (junction 179) : {Trigger1=1;}
  (junction 63) -> (junction 64) : [select_on_num==1]
  (junction 63) -> (junction 65)
  (junction 64) -> (junction 72) : {Trigger1=1;}
  (junction 185) -> (junction 178) : [last_num==2]
  (junction 185) -> (junction 169)
  (junction 178) -> (junction 174) : {Trigger2=1;}
  (junction 65) -> (junction 66) : [select_on_num==2]
  (junction 65) -> (junction 67)
  (junction 66) -> (junction 71) : {Trigger2=1;}
  (junction 169) -> (junction 170) : [last_num==3]
  (junction 169) -> (junction 160)
  (junction 170) -> (junction 175) : {Trigger3=1;}
  (junction 67) -> (junction 68) : [select_on_num==3]
  (junction 67) -> (junction 89)
  (junction 68) -> (junction 70) : {Trigger3=1;}
  (junction 174) -> (junction 175)
  (junction 179) -> (junction 174)
  (junction 175) -> (junction 166)
  (junction 71) -> (junction 70)
  (junction 72) -> (junction 71)
  (junction 70) -> (junction 98)
  (junction 160) -> (junction 159) : [last_num==4]
  (junction 160) -> (junction 161)
  (junction 159) -> (junction 166) : {Trigger4=1;}
  (junction 89) -> (junction 90) : [select_on_num==4]
  (junction 89) -> (junction 91)
  (junction 90) -> (junction 98) : {Trigger4=1;}
  (junction 161) -> (junction 162) : [last_num==5]
  (junction 161) -> (junction 163)
  (junction 162) -> (junction 167) : {Trigger5=1;}
  (junction 91) -> (junction 92) : [select_on_num==5]
  (junction 91) -> (junction 93)
  (junction 92) -> (junction 97) : {Trigger5=1;}
  (junction 163) -> (junction 164) : [last_num==6]
  (junction 163) -> (junction 223)
  (junction 164) -> (junction 165) : {Trigger6=1;}
  (junction 93) -> (junction 94) : [select_on_num==6]
  (junction 93) -> (junction 115)
  (junction 94) -> (junction 96) : {Trigger6=1;}
  (junction 223) -> (junction 217) : [last_num==7]
  (junction 223) -> (junction 227)
  (junction 217) -> (junction 218) : {Trigger7=1;}
  (junction 167) -> (junction 165)
  (junction 166) -> (junction 167)
  (junction 115) -> (junction 116) : [select_on_num==7]
  (junction 165) -> (junction 218)
  (junction 115) -> (junction 117)
  (junction 116) -> (junction 124) : {Trigger7=1;}
  (junction 97) -> (junction 96)
  (junction 98) -> (junction 97)
  (junction 96) -> (junction 124)
  (junction 227) -> (junction 211) : [last_num==8]
  (junction 227) -> (junction 228)
  (junction 211) -> (junction 210) : {Trigger8=1;}
  (junction 117) -> (junction 118) : [select_on_num==8]
  (junction 117) -> (junction 119)
  (junction 118) -> (junction 123) : {Trigger8=1;}
  (junction 228) -> (junction 222) : [last_num==9]
  (junction 228) -> (junction 197)
  (junction 222) -> (junction 224) : {Trigger9=1;}
  (junction 119) -> (junction 120) : [select_on_num==9]
  (junction 119) -> (junction 137)
  (junction 120) -> (junction 122) : {Trigger9=1;}
  (junction 197) -> (junction 204) : [last_num==10]
  (junction 210) -> (junction 224)
  (junction 218) -> (junction 210)
  (junction 197) -> (junction 199)
  (junction 204) -> (junction 208) : {Trigger10=1;}
  (junction 224) -> (junction 208)
  (junction 137) -> (junction 138) : [select_on_num==10]
  (junction 123) -> (junction 122)
  (junction 124) -> (junction 123)
  (junction 137) -> (junction 139)
  (junction 138) -> (junction 143) : {Trigger10=1;}
  (junction 122) -> (junction 143)
  (junction 199) -> (junction 206) : [last_num==11]
  (junction 199) -> (junction 205) : {Trigger12=1;}
  (junction 206) -> (junction 207) : {Trigger11=1;}
  (junction 139) -> (junction 140) : [select_on_num==11]
  (junction 139) -> (junction 141) : {Trigger12=1;}
  (junction 140) -> (junction 142) : {Trigger11=1;}
  (junction 146) -> (junction 205)
  (junction 144) -> (junction 146)
  (junction 207) -> (junction 205)
  (junction 208) -> (junction 207)
  (junction 205) -> (junction 233)
  (junction 142) -> (junction 141)
  (junction 143) -> (junction 142)
  (junction 141) -> (junction 144)
  data: A_D_C input; select_on_num input; last_num input; Trigger1 output single =0; Trigger2 output single =0; Trigger3 output single =0; Trigger4 output single =0; Trigger5 output single =0; Trigger6 output single =0; Trigger7 output single =0; Trigger8 output single =0; Trigger9 output single =0; Trigger10 output single =0; Trigger11 output single =0; Trigger12 output single =0
